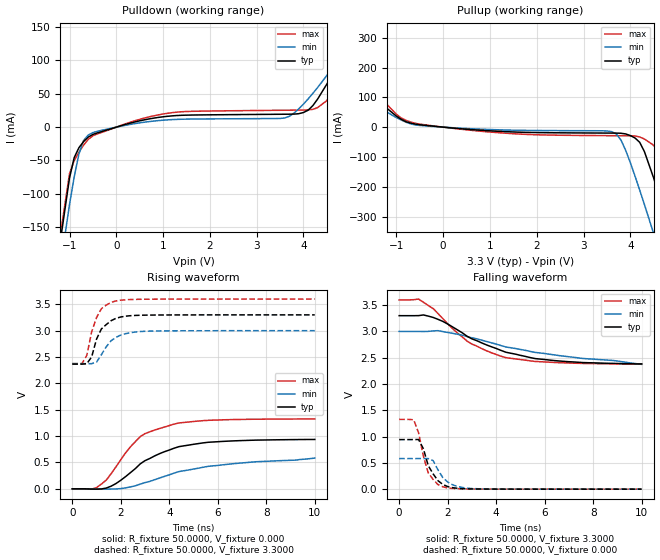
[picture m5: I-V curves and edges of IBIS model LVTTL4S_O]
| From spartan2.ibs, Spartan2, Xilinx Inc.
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|   Model LVTTL4S_O
[Model]   LVTTL4S_O
Model_type   Output
Polarity   Non-Inverting
Vmeas =   1.4000V
Cref =  35.0000pF
Rref =   1.0000M
Vref =  0.000V
C_comp   6.5000pF   5.0000pF   8.0000pF
[Temperature Range]   27.0000   100.0000   0.000
[Voltage Range]   3.3000V   3.0000V   3.6000V
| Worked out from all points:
|   slope of the pulldown table from 0 to 0.495 V, typ, clamps not added: 52.7 ohm
|   slope of the pullup table from 0 to 0.495 V, typ, clamps not added: 72 ohm
|   rising waveform, R_fixture 50.0000, V_fixture 0.000: 20-80 % time 2.01ns typ, 3.45ns min, 1.51ns max; typ from 0 V to 0.937 V
|   rising waveform, R_fixture 50.0000, V_fixture 3.3000: 20-80 % time 564ps typ, 671ps min, 487ps max; typ from 2.37 V to 3.3 V
|   falling waveform, R_fixture 50.0000, V_fixture 3.3000: 20-80 % time 2.73ns typ, 4.31ns min, 2.08ns max; typ from 3.3 V to 2.38 V
|   falling waveform, R_fixture 50.0000, V_fixture 0.000: 20-80 % time 550ps typ, 587ps min, 467ps max; typ from 0.943 V to 0 V
[Pulldown]
| voltage   I(typ)   I(min)   I(max)
-3.3V     -1.286A    -1.273A    -1.29A
-1.5V     -317.7mA   -354.1mA   -304.2mA
-1V       -76.21mA   -116mA     -69.81mA
-800mV    -30.95mA   -40.58mA   -37.74mA
-500mV    -10.89mA   -8.192mA   -12.96mA
1.2V      16.95mA    11.33mA    21.76mA
3.6V      19.37mA    13.78mA    25.36mA
4.1V      25.44mA    42.35mA    25.81mA
4.5V      64.6mA     77.61mA    39.82mA
5.1V      143.3mA    138.1mA    128.1mA
5.3V      171mA      159.5mA    161.3mA
6.6V      348mA      295mA      376.7mA
[Pullup]
| voltage   I(typ)   I(min)   I(max)
-3.3V     354.4mA    271.9mA    429.9mA
-2.7V     272.8mA    207.8mA    331mA
-800mV    18.43mA    17.03mA    23.04mA
3.6V      -19.96mA   -15.22mA   -28.65mA
3.8V      -20.52mA   -43.41mA   -28.84mA
4.2V      -51mA      -211.2mA   -32.92mA
4.5V      -171.4mA   -357.8mA   -61.08mA
4.7V      -272mA     -457.9mA   -116mA
4.9V      -376.2mA   -559mA     -210.3mA
5.1V      -482.2mA   -660.7mA   -313.6mA
5.3V      -589.2mA   -762.8mA   -420.3mA
6.6V      -1.293A    -1.432A    -1.133A
[Ramp]
| variable   typ   min   max
dV/dt_r   0.5622/2.0206n   0.3323/2.9769n   0.7950/1.5333n
dV/dt_f   0.5508/2.7270n   0.3456/3.6283n   0.7320/2.0742n
R_load = 50.0000
[Rising Waveform]
R_fixture = 50.0000
V_fixture = 0.000
| time   V(typ)   V(min)   V(max)
0s        0V         0V         0V
800ps     -4.944mV   227.6uV    -6.08mV
1ns       -5.859mV   -1.95mV    24.41mV
1.4ns     14.65mV    -5.822mV   166.1mV
1.8ns     99.94mV    -1.623mV   416.7mV
2.4ns     307.7mV    36.82mV    798.3mV
2.8ns     472.4mV    89.52mV    989.3mV
4.2ns     770.7mV    298.6mV    1.228V
5.6ns     882.9mV    426.6mV    1.3V
10ns      937mV      583.8mV    1.325V
[Rising Waveform]
R_fixture = 50.0000
V_fixture = 3.3000
V_fixture_min = 3.0000
V_fixture_max = 3.6000
| time   V(typ)   V(min)   V(max)
0s        2.365V     2.374V     2.375V
400ps     2.365V     2.374V     2.375V
600ps     2.373V     2.374V     2.532V
800ps     2.503V     2.374V     2.98V
1ns       2.839V     2.404V     3.247V
1.2ns     3.032V     2.544V     3.417V
1.6ns     3.189V     2.808V     3.536V
1.8ns     3.233V     2.873V     3.563V
3ns       3.294V     2.988V     3.596V
10ns      3.299V     2.999V     3.599V
[Falling Waveform]
R_fixture = 50.0000
V_fixture = 3.3000
V_fixture_min = 3.0000
V_fixture_max = 3.6000
| time   V(typ)   V(min)   V(max)
0s        3.3V       3V         3.6V
800ps     3.301V     3V         3.616V
1ns       3.314V     2.999V     3.556V
1.6ns     3.231V     3.015V     3.342V
2.8ns     2.909V     2.903V     2.817V
3.6ns     2.744V     2.809V     2.633V
4.4ns     2.605V     2.705V     2.502V
5.6ns     2.485V     2.602V     2.43V
6.6ns     2.438V     2.541V     2.406V
10ns      2.382V     2.374V     2.38V
[Falling Waveform]
R_fixture = 50.0000
V_fixture = 0.000
| time   V(typ)   V(min)   V(max)
0s        943.3mV    581.6mV    1.327V
600ps     943.5mV    581.6mV    1.32V
800ps     944.6mV    581.7mV    1.073V
1ns       768.5mV    581.9mV    624.7mV
1.2ns     447mV      582.5mV    311.4mV
1.4ns     292mV      543.9mV    184.9mV
1.8ns     90.22mV    221.4mV    44.92mV
2.2ns     28.84mV    83.5mV     14.21mV
3ns       4.552mV    12.04mV    3.466mV
10ns      359.8uV    293.3uV    372.9uV
